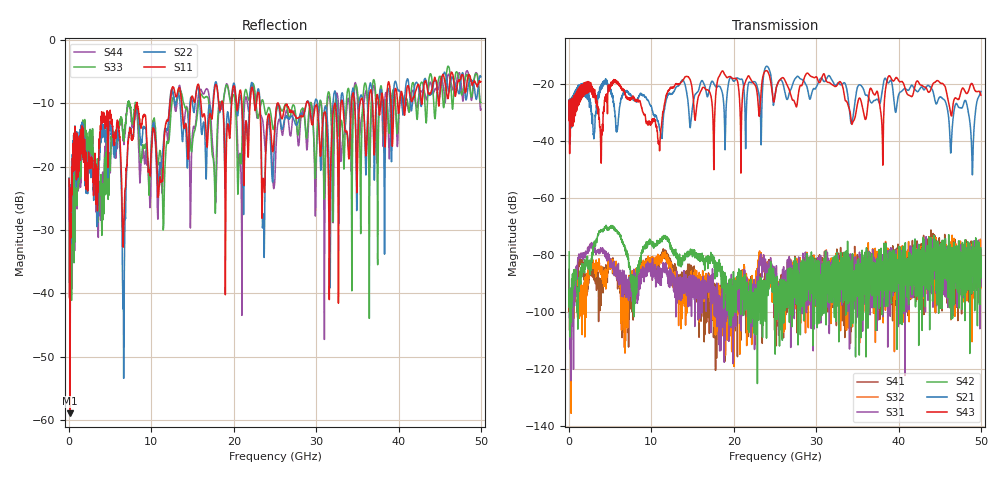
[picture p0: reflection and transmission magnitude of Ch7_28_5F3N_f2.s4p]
!Agilent Technologies,N5247A,US51170199,A.09.90.13
!Agilent N5247A: A.09.90.13
!Date: Wednesday, December 09, 2015 09:38:09
!Correction: S11(Full 4 Port(1,2,3,4))
!S12(Full 4 Port(1,2,3,4))
!S13(Full 4 Port(1,2,3,4))
!S14(Full 4 Port(1,2,3,4))
!S21(Full 4 Port(1,2,3,4))
!S22(Full 4 Port(1,2,3,4))
!S23(Full 4 Port(1,2,3,4))
!S24(Full 4 Port(1,2,3,4))
!S31(Full 4 Port(1,2,3,4))
!S32(Full 4 Port(1,2,3,4))
!S33(Full 4 Port(1,2,3,4))
!S34(Full 4 Port(1,2,3,4))
!S41(Full 4 Port(1,2,3,4))
!S42(Full 4 Port(1,2,3,4))
!S43(Full 4 Port(1,2,3,4))
!S44(Full 4 Port(1,2,3,4))
!S4P File: Measurements: <S11,S12,S13,S14>,
!<S21,S22,S23,S24>,
!<S31,S32,S33,S34>,
!<S41,S42,S43,S44>:
# Hz S  dB  R 50
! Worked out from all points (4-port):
!   3201 points, 10 MHz to 50 GHz, reference 50 ohm
!   strongest paths, dB at 10 MHz, 12.51 GHz, 25 GHz, 37.5 GHz, 50 GHz:
!     S43: -33.0, -21.3, -24.2, -23.6, -24.1
!     S21: -32.5, -23.5, -24.2, -25.7, -22.8
!     S42: -78.9, -78.0, -90.8, -85.6, -77.7
!     S31: -92.3, -86.9, -88.3, -87.8, -83.7
!     S32: -85.8, -84.9, -92.9, -90.0, -86.2
!     S41: -85.1, -83.6, -96.7, -81.9, -87.0
!   lowest |S11| = -58.9 dB at 135 MHz (marker M1), VSWR 1.00, Z = 50 + j0.113 ohm
!   |S11| at or under -10 dB: start of sweep to 8.238 GHz; 8.267 GHz to 12.25 GHz (3.978 GHz wide, 38.8 % of centre); 29.06 GHz to 33.02 GHz (3.962 GHz wide, 12.8 % of centre)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
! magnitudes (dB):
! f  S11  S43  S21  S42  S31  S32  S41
! 10 MHz  -22.0  -33.0  -32.5  -78.9  -92.3  -85.8  -85.1
! 135 MHz  -58.9  -32.2  -32.8  -95.9  -96.5  -96.8  -97.4
! 24.04 GHz  -13.3  -15.6  -13.9  -93.4  -89.4  -86.8  -86.5
! 37.99 GHz  -8.4  -34.6  -23.2  -91.6  -86.3  -89.2  -84.3
! 38.86 GHz  -6.9  -17.3  -19.5  -83.0  -93.0  -83.2  -81.1
! 48.95 GHz  -7.2  -20.1  -51.3  -85.5  -78.1  -80.1  -87.8
! 50 GHz  -6.6  -24.1  -22.8  -77.7  -83.7  -86.2  -87.0
